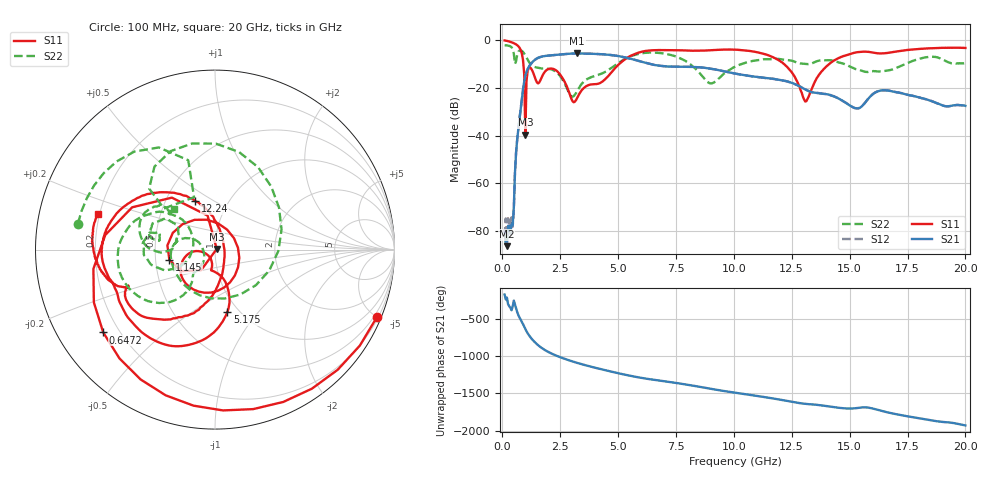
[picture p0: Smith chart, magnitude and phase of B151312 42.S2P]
!  2-Port S-parameters saved by WinCal
! VAR MeasName=S-Parameters (CALIBRATED_DATA) read from VNA (N5244A)
! VAR MeasDate=12/8/2015 5:47:14 PM
! VAR NAME=B151312 42
! VAR FILENAME=B151312 42.S2P
! VAR DATE=12/8/2015 5:47:14 PM
! VAR PHYS_PORTS=1,2
# Hz S DB R 50
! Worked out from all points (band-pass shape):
!   401 points, 100 MHz to 20 GHz, reference 50 ohm
!   highest |S21| = -5.65 dB at 3.234 GHz (marker M1); lowest = -86.3 dB at 199.5 MHz (marker M2)
!   |S21| within 3 dB of the highest: 1.365 GHz to 5.847 GHz (4.482 GHz wide, 124 % of centre)
!   lowest |S11| = -39.7 dB at 995.5 MHz (marker M3), VSWR 1.02, Z = 51 + j0.377 ohm
!   |S11| at or under -10 dB: 909 MHz to 5.055 GHz (4.146 GHz wide, 139 % of centre); 12.16 GHz to 14.12 GHz (1.962 GHz wide, 14.9 % of centre)
!   |S22| runs from -23.7 to -2.2 dB; largest |S21 - S12| = 0.0021
!   S11 on the Smith chart (normalised r, x): 100 MHz: 0.29, -4.99; 647.2 MHz: 0.14, -0.32; 1.145 GHz: 0.59, -0.07; 5.175 GHz: 0.89, -0.70; 12.24 GHz: 0.70, +0.41; 20 GHz: 0.19, +0.15
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1e8  -0.20 -22.6  -79.74 -176.1  -81.91 171.9  -2.19 169.3
1.995e8  -0.38 -44.4  -86.29 142.6  -82.57 74.0  -2.28 158.2
3.985e8  -0.94 -87.2  -77.07 -26.5  -74.25 -42.5  -3.01 129.5
6.4725e8  -2.21 -143.5  -41.22 -54.3  -41.23 -54.4  -6.01 137.2
9.955e8  -39.67 20.9  -14.97 82.6  -14.97 82.6  -6.55 48.2
1.14475e9  -11.69 -167.3  -11.29 1.3  -11.29 1.3  -9.05 -1.4
1.44325e9  -16.62 83.6  -8.05 -106.4  -8.05 -106.4  -11.43 -108.4
1.7915e9  -13.95 -65.3  -6.78 169.5  -6.77 169.5  -11.96 -157.8
2.3885e9  -13.25 -152.2  -6.16 77.7  -6.16 77.7  -13.89 163.3
3.23425e9  -24.25 -110.5  -5.65 -12.2  -5.65 -12.2  -21.31 -136.4
3.43325e9  -20.98 -100.3  -5.67 -30.1  -5.66 -30.0  -18.32 -131.2
4.22925e9  -17.98 -88.7  -5.92 -93.9  -5.92 -94.0  -14.30 -129.7
5.1745e9  -9.02 -78.8  -7.04 -162.3  -7.02 -162.2  -8.61 -129.5
6.7665e9  -4.22 -131.5  -10.75 111.7  -10.74 111.6  -5.41 178.6
8.9555e9  -4.30 -164.6  -11.96 3.1  -11.93 2.7  -18.13 165.6
1.005e10  -4.05 175.9  -14.05 -52.1  -14.04 -52.3  -11.14 -156.2
1.2239e10  -10.74 112.0  -17.16 -158.4  -17.20 -158.4  -8.34 168.1
1.308475e10  -25.75 14.5  -20.71 158.9  -20.71 159.1  -10.03 167.8
1.338325e10  -19.95 -61.7  -21.91 151.6  -21.86 151.5  -9.74 171.2
1.45275e10  -7.55 -116.3  -24.53 106.2  -24.50 105.9  -9.43 150.7
1.67165e10  -5.33 -157.3  -21.29 39.0  -21.18 38.4  -12.64 177.2
2e10  -3.33 162.8  -27.56 -130.9  -27.66 -131.3  -9.89 135.1
